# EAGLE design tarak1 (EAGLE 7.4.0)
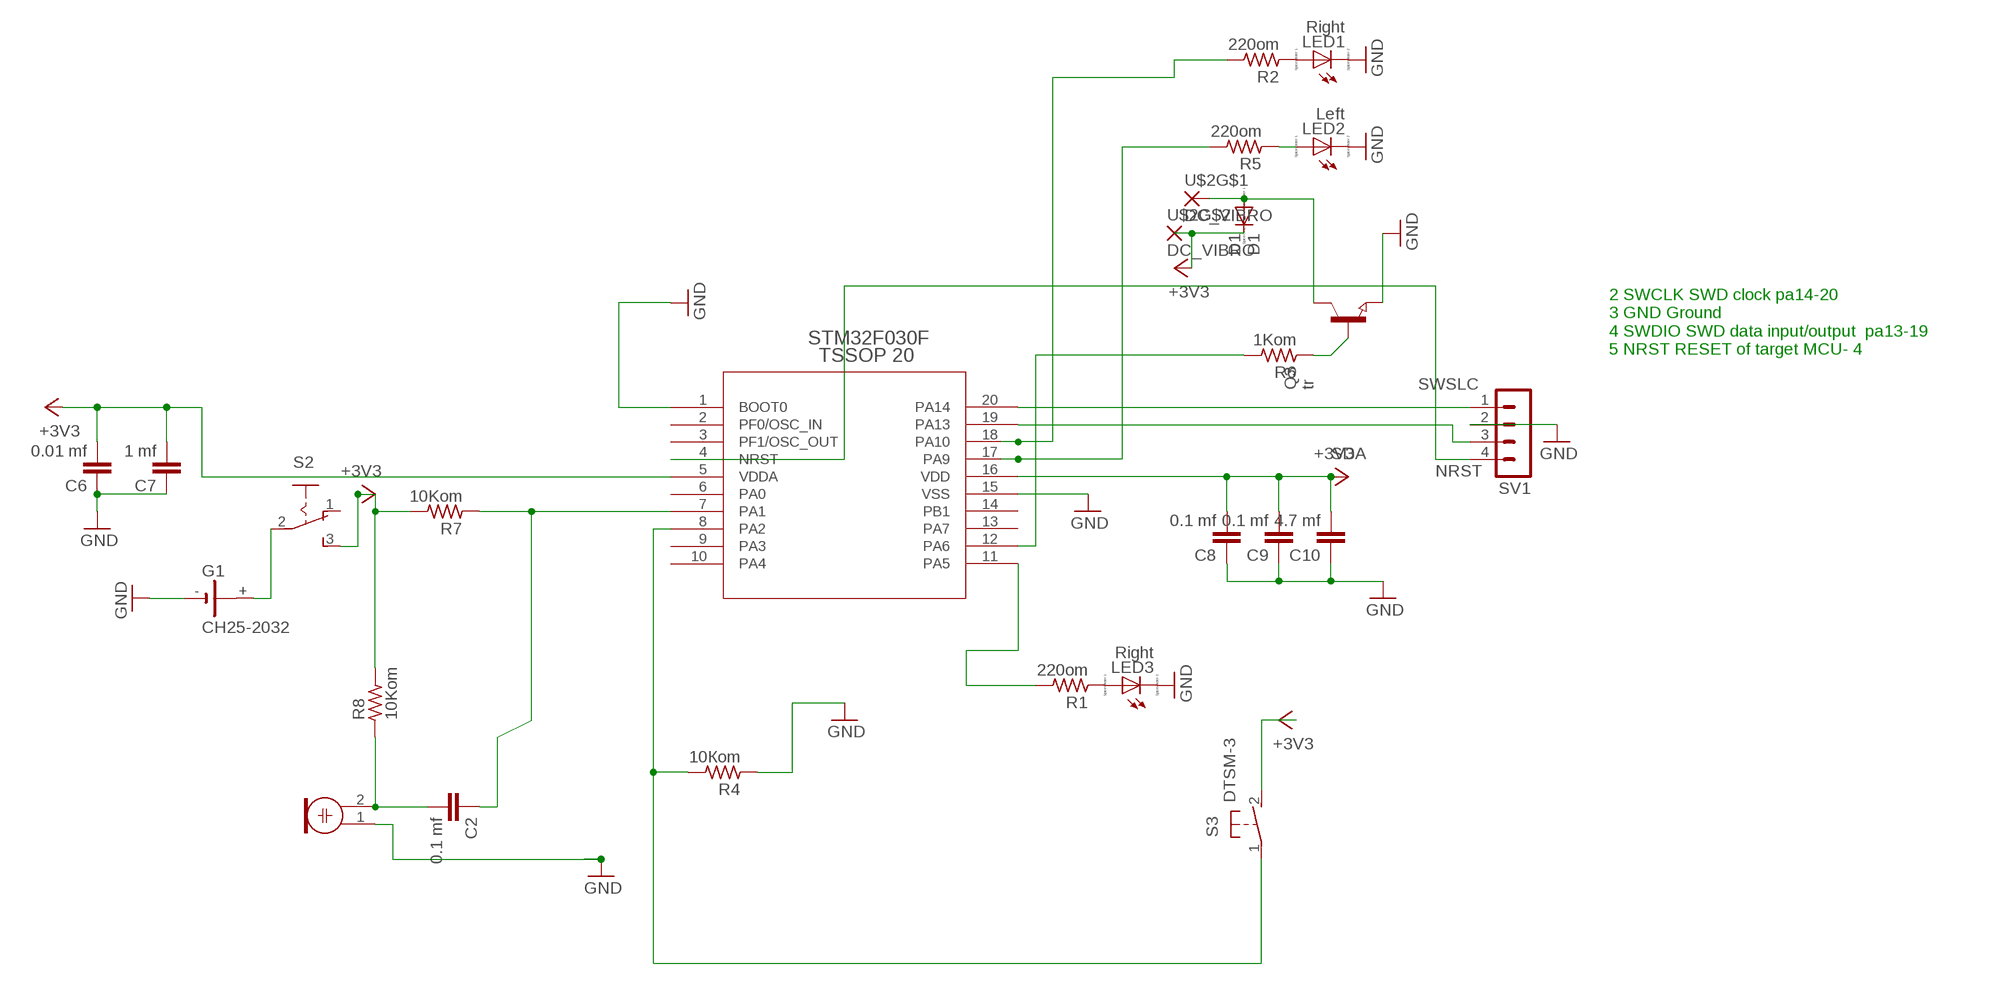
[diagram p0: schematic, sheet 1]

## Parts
C2  0.1 mf  CAP1206  [1206]
C6  0.01 mf  CAP1206  [1206]
C7  1 mf  CAP1206  [1206]
C8  0.1 mf  CAP1206  [1206]
C9  0.1 mf  CAP1206  [1206]
C10  4.7 mf  CAP1206  [1206]
D1  D1  DIODE-MINIMELF  [MINIMELF]
G1  CH25-2032  [CH25-2032]
LED1  Right  LED_ESML0603  [LED_SML0603]
LED2  Left  LED_ESML0603  [LED_SML0603]
LED3  Right  LED_E  [LED_1206]
M1  ELECTRET_MICROPHON-F6050AP  [F6050AP]
Q3  tr  NPN-TRANSISTOR_SOT23  [SOT23]
R1  220om  STM32F050F-BASE_R_1206  [STM32F050F-BASE_R1206]
R2  220om  STM32F050F-BASE_R_1206  [STM32F050F-BASE_R1206]
R4  10Кom  STM32F050F-BASE_R_1206  [STM32F050F-BASE_R1206]
R5  220om  STM32F050F-BASE_R_1206  [STM32F050F-BASE_R1206]
R6  1Kom  STM32F050F-BASE_R_1206  [STM32F050F-BASE_R1206]
R7  10Kom  STM32F050F-BASE_R_1206  [STM32F050F-BASE_R1206]
R8  10Kom  STM32F050F-BASE_R_1206  [STM32F050F-BASE_R1206]
S2  SS12F27  [SS12F27]
S3  DTSM-3  [DTSM-3]
SV1  MA04-1  [MA04-1]
U$1  STM32F030F  [STM32F050F-BASE_TSSOP20]
U$2  DC_VIBRO  [DC_VIBRO]

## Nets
+3V3: C6.2 C7.2 C8.2 C9.2 C10.2 D1.C R7.2 R8.2 S2.3(S) S3.2 U$1.5(VDDA) U$1.16(VDD) U$2.P$3
GND: C6.1 C7.1 C8.1 C9.1 C10.1 G1.- LED1.C LED2.C LED3.C M1.1 Q3.2(E) R4.1 SV1.2 U$1.1(BOOT0) U$1.15(VSS)
N$1: D1.A Q3.3(C) U$2.P$1
N$2: R6.2 U$1.12(PA6)
N$3: R1.2 U$1.11(PA5)
N$4: G1.+ S2.2(P)
N$5: R5.2 U$1.17(PA9)
N$6: LED1.A R2.1
N$7: LED3.A R1.1
N$17: LED2.A R5.1
N$22: R2.2 U$1.18(PA10)
N$26: R4.2 S3.1 U$1.8(PA2)
N$28: Q3.1(B) R6.1
N$43: C2.2 M1.2 R8.1
N$46: C2.1 R7.1 U$1.7(PA1)
NRST: SV1.4 U$1.4(NRST)
SDA: SV1.3 U$1.19(PA13)
SWSLC: SV1.1 U$1.20(PA14)
Unconnected: S2.1(O) U$1.2(PF0/OSC_IN) U$1.3(PF1/OSC_OUT) U$1.6(PA0) U$1.9(PA3) U$1.10(PA4) U$1.13(PA7) U$1.14(PB1)

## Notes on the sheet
- 2 SWCLK SWD clock pa14-20 
  3 GND Ground 
  4 SWDIO SWD data input/output  pa13-19 
  5 NRST RESET of target MCU- 4

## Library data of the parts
C2 C6-C10 = SparkFun-Capacitors:CAP: Capacitor
D1 = diode:DIODE-: DIODE
G1 = tarak:CH25-2032: LI BATTERY Varta
LED1-LED3 = eagle-ltspice:LED_E: LED; SPICEMODEL: NONE; SPICEPREFIX: D; SPICETYPE: diode
M1 = microphon:ELECTRET_MICROPHON-: Electret Condenser Microphone
Q3 = semicon-smd-ipc:NPN-TRANSISTOR_: NPN TRANSISTOR
R1 R2 R4-R8 = clockclock1:STM32F050F-BASE_R_: RESISTOR
S2 = tarak:SS12F27: SLIDING SWITCH Distributor Buerklin, 11G810
S3 = switch-tact:DTSM-3
SV1 = con-lstb:MA04-1: PIN HEADER; OC_FARNELL: unknown; OC_NEWARK: unknown
U$1 = clockclock1:STM32F030F: STM32F050F4P6
U$2 = tarak:DC_VIBRO

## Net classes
0 default: width 0.254 mm, drill 0.254 mm, clearance 0.2 mm

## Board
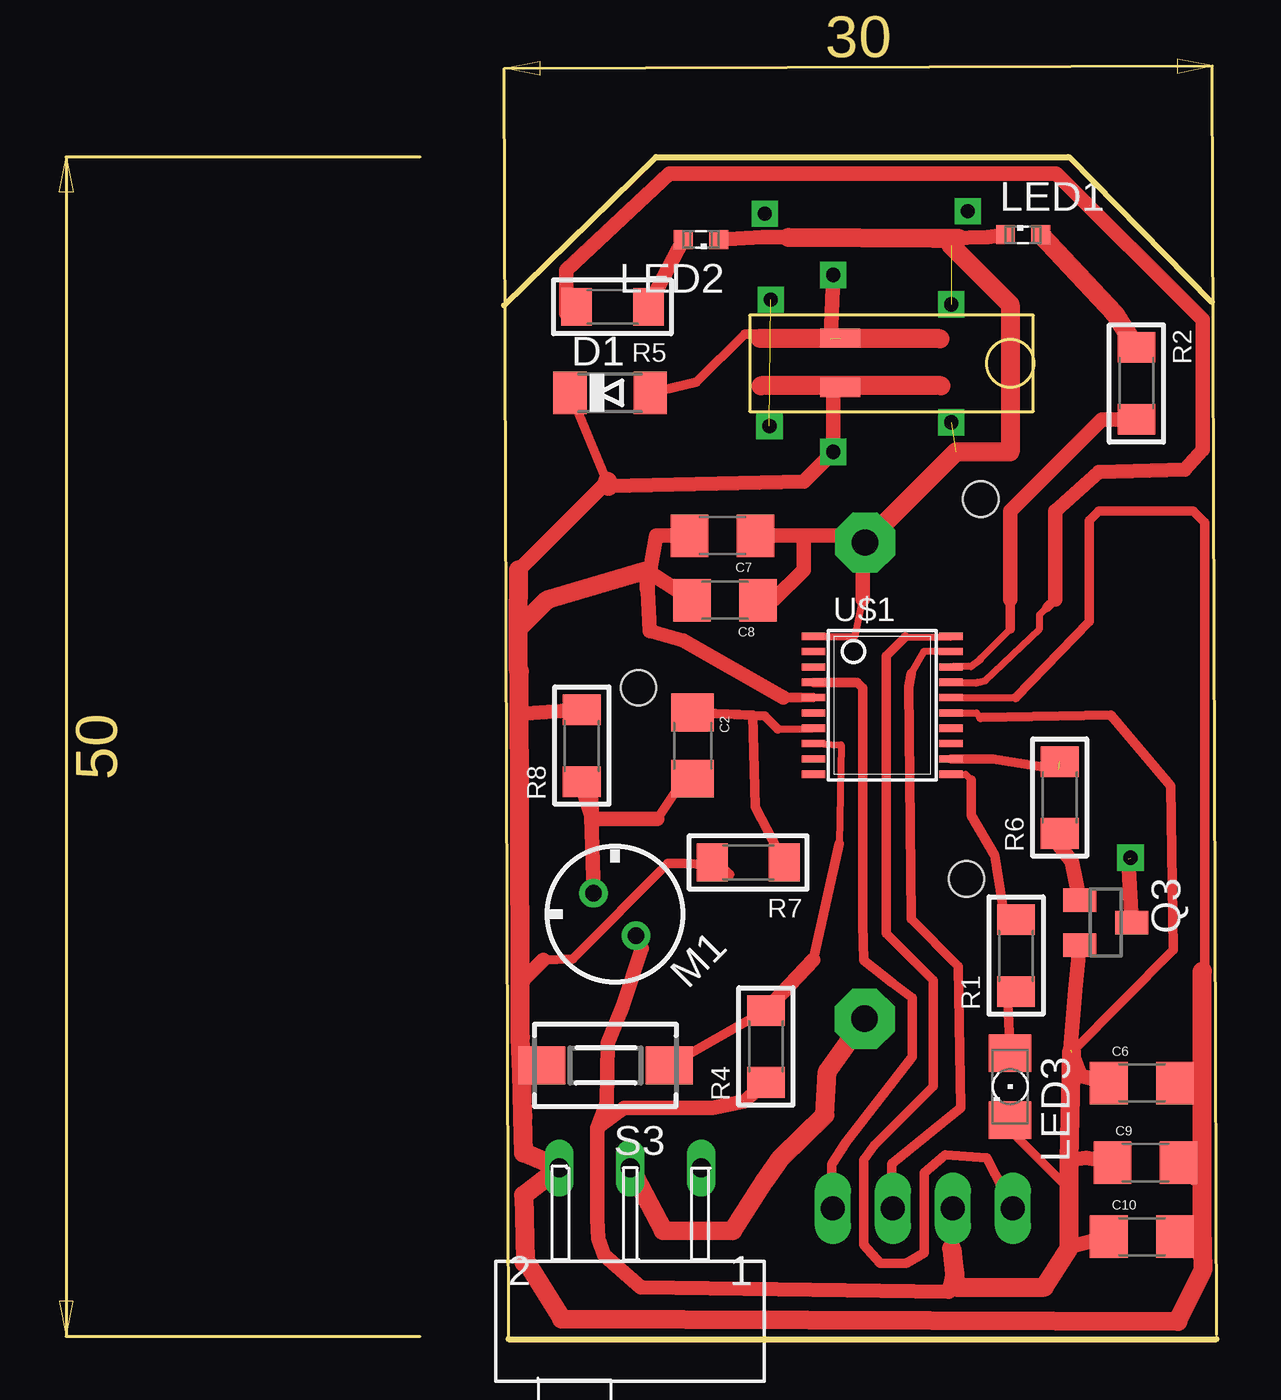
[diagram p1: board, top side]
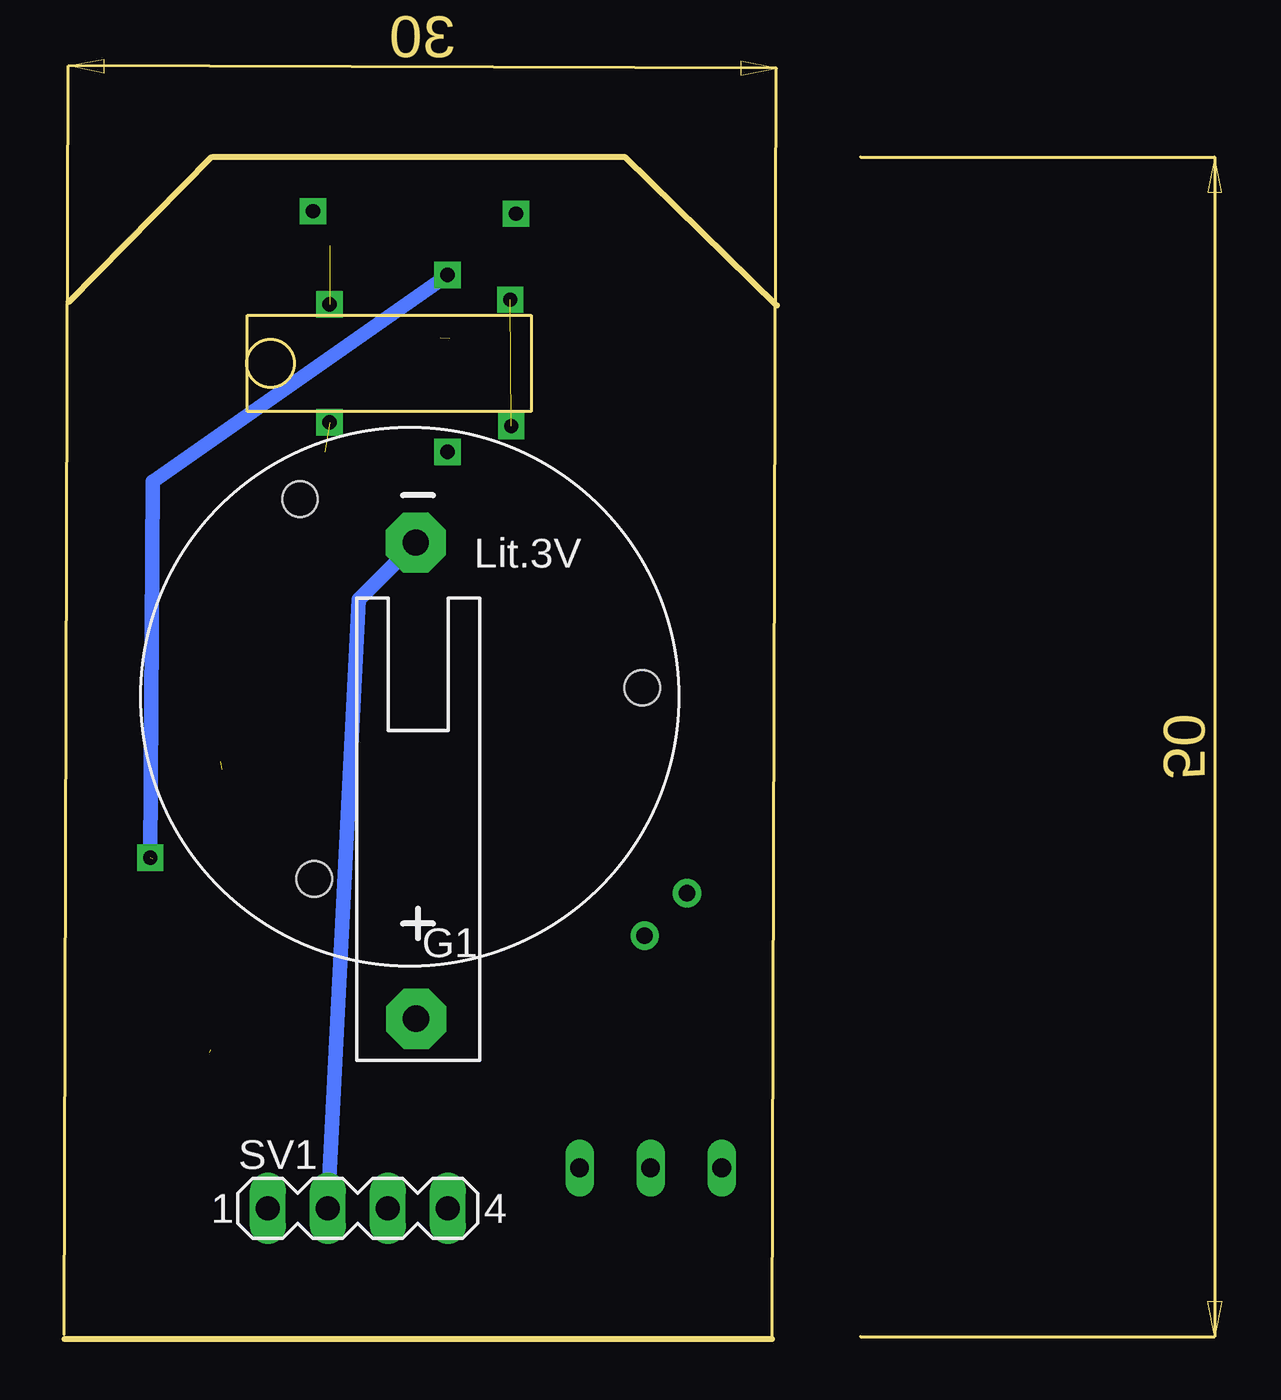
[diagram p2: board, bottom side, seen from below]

Size 49.05 x 54.25 mm. Coordinates in mm from the lower left corner, seen from the top.
Outline: 19.05,0 49.04,0
Outline: 25.3,50.1 42.74,50.1
Outline: 25.28,50.08 18.85,43.8
Outline: 42.82,50.08 48.85,43.95
Copper layers (1*16): Top 0.035mm / dielectric 1.5mm / Bottom 0.035mm
Design rules "default *": minimum track width 8mil, minimum drill 10mil, track to track 4mil, track to pad 4mil, pad to pad 4mil, via to via 4mil, smd to smd 4mil, copper to edge 4mil, drill to drill 4mil, minimum pad ring 8mil, minimum via ring 8mil, stop-mask expansion 4mil, vias tented up to drill 0mil, thermal gap 10mil

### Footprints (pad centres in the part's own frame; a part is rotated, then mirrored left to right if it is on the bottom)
1206 = smd 1.6 x 1.8: 1 -1.4,0; 2 1.4,0
MINIMELF = smd 1.4 x 1.8: A 1.7,0; C -1.7,0
CH25-2032 = drill 1.118 pad 2.54 octagon: + -0.08,-14.025; - -0.1,6.155 | hole 1.5: -5,8; 9.5,0; -4.4,-8.1
LED_SML0603 = smd 0.8 x 0.8: A 0.75,0; C -0.75,0
LED_1206 = smd 1.6 x 1.803: A -1.422,0; C 1.422,0
F6050AP = drill 0.7 pad 1.2: 1 0,1.27; 2 0,-1.27
SOT23 = smd 1 x 1.4: 1 -0.95,-1.1; 2 0.95,-1.1; 3 0,1.1
STM32F050F-BASE_R1206 = smd 1.3 x 1.6: 1 -1.524,0; 2 1.524,0
SS12F27 = drill 0.8 long: 1 -3.01,-6.5; 2 0,-6.5; 3 3.01,-6.5
DTSM-3 = smd 2 x 1.6: 1 -2.7,0; 2 2.7,0
MA04-1 = drill 1.016 long: 1 -3.81,0; 2 -1.27,0; 3 1.27,0; 4 3.81,0
STM32F050F-BASE_TSSOP20 = smd 0.305 x 0.991: 1 -2.925,-2.918; 2 -2.275,-2.918; 3 -1.625,-2.918; 4 -0.975,-2.918; 5 -0.325,-2.918; 6 0.325,-2.918; 7 0.975,-2.918; 8 1.625,-2.918; 9 2.275,-2.918; 10 2.925,-2.918; 11 2.925,2.918; 12 2.275,2.918; 13 1.625,2.918; 14 0.975,2.918; 15 0.325,2.918; 16 -0.325,2.918; 17 -0.975,2.918; 18 -1.625,2.918; 19 -2.275,2.918; 20 -2.925,2.918
DC_VIBRO = smd 0.813 x 1.676: P$1 -1.07,-2.2; P$3 1.03,-2.2

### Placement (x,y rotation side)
C2  26.85,25.15 270 top
C6  45.88,10.85 0 top
C7  28.11,34.05 180 top
C8  28.22,31.32 180 top
C9  46.03,7.48 0 top
C10  45.88,4.34 0 top
D1  23.35,40.1 0 top
G1  34.05,27.6 0 bottom
LED1  40.85,46.8 0 top
LED2  27.2,46.6 180 top
LED3  40.3,10.7 270 top
M1  23.55,18 225 top
Q3  44.35,17.65 270 top
R1  40.55,16.25 90 top
R2  45.65,40.5 270 top
R4  29.95,12.4 90 top
R5  23.45,43.75 180 top
R6  42.4,22.95 90 top
R7  29.2,20.2 180 top
R8  22.15,25.15 90 top
S2  24.2,0.75 180 top
S3  23.15,11.6 180 top
SV1  36.6,5.54 0 bottom
U$1  34.88,26.86 270 top
U$2  35.3,41.35 270 top

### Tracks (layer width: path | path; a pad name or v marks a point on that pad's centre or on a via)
+3V3  (via drill 0.6)
  Top 0.305: S3.2 19.94,11.6 19.61,11.27 | U$1.16 40.53,27.19
  Top 0.406: U$1.5 30.69,27.19 | 40.53,27.19 43.65,30.4 43.65,34.7 44.05,35.1 48.05,35.1 48.55,34.6 48.55,15.22 48.43,15.1 | 48.43,4.32 48.27,4.32 47.8,3.85 | D1.C 23.29,36.15 | C6.2 47.73,10.55 48.43,9.85 | C9.2 48.1,6.68 48.43,6.55 | C10.2 48.34,3.94 48.44,3.84 | 20.52,16.08 21.77,16.12 25.8,20.15 26.5,20.15 27.8,20.1 28.1,20 28.42,19.7 R7.2
  Top 0.61: 30.69,27.19 26.45,29.6 25.02,30 24.9,32.57 | U$2.P$3 33.02,40.32 32.8,40.1 v32.8,37.6 31.55,36.35 23.29,36.15 | 23.23,36.35 19.48,32.6 | C7.2 25.3,34.05 24.9,31.82 24.9,32.57 | C8.2 24.9,32.57 | 19.45,28.4 19.47,26.5 R8.2 | 20.52,16.08 19.54,15.1
  Top 0.813: 19.46,30.11 19.45,28.4 19.5,28.3 19.54,15.1 19.55,12.8 19.61,11.27 19.65,9.5 19.65,9.4 19.69,7.89 S2.3 19.69,6.1 19.76,3.33 | 19.46,30.11 19.48,32.6 | 19.7,3.25 19.76,3.33 | 19.76,3.33 21.3,0.85 47.4,0.75 48.45,2.9 48.44,3.84 48.43,4.32 48.43,6.55 48.43,9.85 48.43,15.1 48.43,15.58 48.45,15.6 | 23.29,36.15 23.23,36.35 | 19.46,30.11 20.67,31.32 24.9,32.57
GND  (via drill 0.6)  (3 unrouted)
  Top 0.305: U$1.1 33.73,29.79 34.05,31.35 | U$1.15 38.87,26.54 39.05,26.35
  Top 0.406: 39.05,26.35 44.55,26.45 47.1,23.45 47.2,16.5 42.9,12.15 | 33.86,34.05 G1.- | C8.1 30.27,31.32 | 24.45,16.8 24.7,16.55 | LED3.C 40.37,8.78 42.8,6.35
  Top 0.61: 37.7,46.65 39.35,46.7 LED1.C | R4.1 29.03,10.08 27.7,9.8 23.95,9.8 22.8,8.95 | 22.8,8.95 22.8,5.1 22.85,4.25 23.1,3.55 24.65,2.2 37.7,2 37.92,2.98 | LED2.C 29.8,46.7 30.9,46.7 | 22.8,8.95 23.2,10 23.25,12.55 23.39,12.91 23.86,14.05 24.7,16.55 | G1.- 34.05,33.66 34.05,31.35 | 42.85,12.25 43.05,14.8 Q3.2 | SV1.2 37.82,3.83 | C7.1 31.55,34.05 | 31.55,34.05 33.86,34.05 | 30.27,31.32 31.55,32.6 31.55,34.05 | C6.1 43.3,11.15 42.9,12.15 | C9.1 43.52,7.68 42.8,7.6 | C10.1 42.89,3.94 42.8,3.85 | M1.1 24.45,16.8
  Top 0.813: 37.92,2.98 38,2.2 | 38,2.2 41.75,2.2 42.8,3.85 42.8,6.35 42.8,7.6 42.9,12.15 | 30.9,46.7 37.05,46.65 37.7,46.65 38.1,46.65 37.8,46.35 40.3,43.85 40.3,37.6 38,37.6 G1.- | 37.82,3.83 38,2.2
  Bottom 0.61: SV1.2 36.57,31.34 G1.-
  other vias: 37.8,43.85 37.8,38.85
N$1  (via drill 0.6)  (2 unrouted)
  Top 0.406: D1.A 27,40.55 29.05,42.6 31.41,42.6 29.7,42.4
  Top 0.61: Q3.3 45.3,20.35 | v32.8,45.1 32.7,42.41 29.7,42.4
  Top 0.813: 37.32,42.4 29.7,42.4
  Bottom 0.61: v45.4,20.4 45.3,36.35 v32.8,45.1
N$2  (1 unrouted)
  Top 0.406: U$1.12 39.56,24.59 42.35,24.15
N$3
  Top 0.305: U$1.11 38.41,23.94 38.65,23.7
  Top 0.406: 38.65,23.7 38.65,22.2 39.65,20.5 40.05,17.97 R1.2
N$4
  Top 0.813: S2.2 25.6,4.6 28.55,4.59 29.9,6.7 30.6,7.7 32.45,9.5 32.55,11.35 G1.+
N$5
  Top 0.305: U$1.17 38.91,27.84 38.85,27.8 39.25,27.9 41.55,30.1 41.55,30.7 41.85,31
  Top 0.406: 42.2,31.35 41.85,31
  Top 0.61: R5.2 21.5,43.45 21.5,45.3 25.85,49.4 42.25,49.4 48.45,43.2 48.45,37.7 47.7,36.85 44.05,36.75 42.2,35.1 42.2,31.35
N$6
  Top 0.813: LED1.A 44.7,43.47 R2.1
N$7
  Top 0.406: LED3.A 40.2,14.28 R1.1
N$8  (via drill 0.6)
  other vias: 29.9,47.7
N$9  (via drill 0.6)
  other vias: 38.5,47.8
N$11  (via drill 0.6)  (1 unrouted)
  other vias: 30.15,44.05 30.1,38.7
N$17
  Top 0.61: LED2.A 25.2,44.22 R5.1
N$18
  Top 0.813: 37.37,40.4 29.75,40.4
N$22
  Top 0.305: 40.3,30.1 39.05,28.85 39.05,28.8 38.65,28.5 37.88,28.5 U$1.18
  Top 0.406: 40.3,31.35 40.3,30.1
  Top 0.61: R2.2 44.18,38.98 40.3,35.1 40.3,31.35
N$26
  Top 0.305: U$1.8 33.14,25.19 33.05,21
  Top 0.406: S3.1 R4.2 | 33.05,21 31.95,16.07
  Top 0.61: 31.95,16.07 R4.2
N$28
  Top 0.406: R6.1 42.23,21.43
  Top 0.61: 42.23,21.43 41.95,21.45 42.9,20.25 Q3.1
N$43
  Top 0.406: 25.35,22.05 26.15,23.25 C2.2
  Top 0.61: R8.1 22.17,23.33 22.6,22.05 | 22.6,22.05 22.5,23.45 M1.2 | 22.6,22.05 25.35,22.05
N$46
  Top 0.305: 30.45,25.85 31.93,25.85 U$1.7
  Top 0.406: 30.45,25.85 29.9,26.4 C2.1 29.4,26.45 29.5,22.55 R7.1
NRST
  Top 0.406: U$1.4 33.81,27.84 34.05,27.6 34.05,17.6 34.1,16.05 35.3,15.1 36.15,14.45 36.15,11.95 33.35,8.35 32.75,7.4 SV1.4
SDA
  Top 0.305: 36.1,28.2 36.65,29.15 37.78,29.15 U$1.19
  Top 0.406: SV1.3 35.28,7.43 38.2,9.8 38.1,15.8 36.1,17.8 36,27.65 36.1,28.2
SWSLC
  Top 0.305: 35.85,29.75 37.76,29.75 U$1.20
  Top 0.406: SV1.1 39.31,7.69 37.55,7.8 36.65,7.05 36.65,3.65 35.9,3.2 34.8,3.2 34.1,4 34.1,7.6 34.55,8.2 37.05,10.7 37.05,15.2 35.05,17.2 35.05,28.95 35.85,29.75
